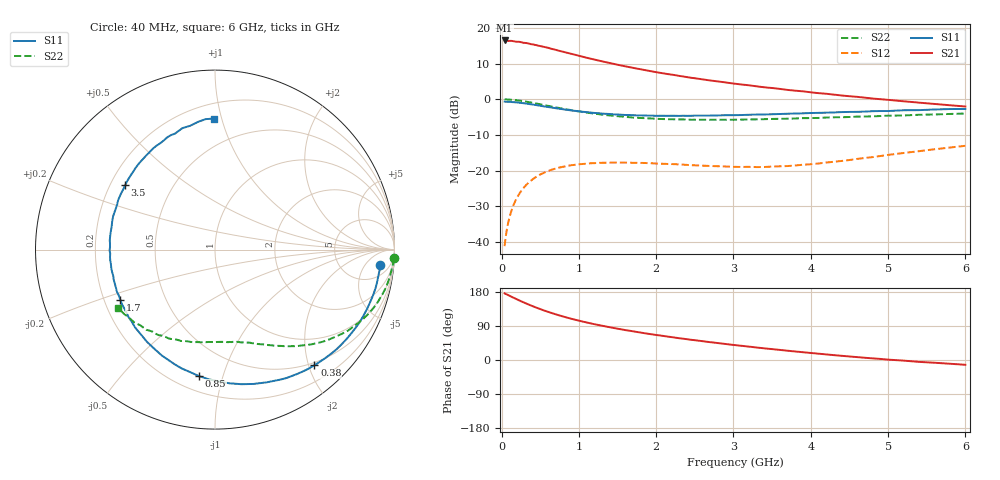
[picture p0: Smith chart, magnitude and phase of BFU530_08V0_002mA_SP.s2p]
! Filename:  P:\Prog\Test\Noise\ATS_data\Testdata_Net\03 Spar\BFU530_APG2013_40_A05_08p0V_002mA_SP_CM01_D.s2p
! Date/Time: Fri 26/Apr/2013 13:03:14
! BFU530_APG2013_40_A05_08p0V_1to25mA_SP_CM01_Bias2_R.s2p
! MDIF S-parameter v. bias file
! BFU530_APG2013_40_A05_08p0V_1to25mA_SP_CM01
! Date/time Wed Apr 24 16:58:28 2013
! VAR V_out= 8.0000
! VAR I_out= 1.9900
! VAR V_in= 0.7959
! VAR I_in= 0.0207
! Device data file deembeded for feedlines and parallel
! Original file: \03 Spar\BFU530_APG2013_40_A05_08p0V_002mA_SP_CM01_R.s2p
! Feed-files: PR047V01_250413_Feed1.s2p, PR047V01_250413_Feed2.s2p
! Parallel-file: PR047V01_250413_Par.s2p
# MHz S MA R 50
!  Freq-MHz  S11-mag  S11-arg  S21-mag  S21-arg  S12-mag  S12-arg  S22-mag  S22-arg
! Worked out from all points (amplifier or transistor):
!   98 points, 40 MHz to 6 GHz, reference 50 ohm
!   highest |S21| = 16.5 dB at 40 MHz (marker M1)
!   |S21| within 3 dB of that: start of sweep to 763.9 MHz
!   unconditionally stable (mu >= 1): 2.894 GHz to 4.763 GHz
!   at 300 MHz: K = 0.11, MSG = 20.1 dB, |S12| = -24.5 dB
!   at 1.6 GHz: K = 0.54, MSG = 13.5 dB, |S12| = -17.8 dB
!   at 6 GHz: K = 0.80, MSG = 5.5 dB, |S12| = -13.1 dB
!   S11 on the Smith chart (normalised r, x): 40 MHz: 10, -13; 380 MHz: 0.45, -2.10; 850 MHz: 0.29, -0.84; 1.7 GHz: 0.27, -0.23; 3.5 GHz: 0.26, +0.30; 6 GHz: 0.30, +0.94
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40  0.9255 -5.5  6.669 175.9  0.008713 86.6  0.9958 -2.9
50  0.9245 -6.8  6.667 174.5  0.0108 86.0  0.9954 -3.6
70  0.9218 -9.3  6.628 172.9  0.01507 84.1  0.9926 -5.3
120  0.9167 -16.2  6.591 167.8  0.02557 80.0  0.9848 -9.0
240  0.8904 -32.0  6.353 156.2  0.0491 70.5  0.9537 -17.7
320  0.868 -42.2  6.143 149.0  0.06293 64.6  0.9245 -23.1
380  0.8498 -49.3  5.919 143.9  0.07216 60.5  0.8997 -26.8
460  0.824 -58.7  5.7 137.5  0.08327 55.6  0.8684 -31.3
600  0.7787 -74.0  5.27 127.2  0.09837 47.8  0.8086 -38.3
750  0.7348 -88.4  4.76 117.6  0.1103 40.8  0.7526 -44.5
850  0.7099 -97.3  4.473 111.7  0.116 36.9  0.7181 -48.1
1050  0.667 -113.2  3.944 101.4  0.1237 30.2  0.6606 -54.5
1200  0.6431 -123.7  3.603 94.5  0.1271 26.2  0.6273 -58.5
1350  0.6248 -133.0  3.307 88.4  0.1288 23.0  0.5997 -62.0
1700  0.5973 -151.9  2.757 75.8  0.1284 17.6  0.5537 -69.5
2050  0.5868 -167.8  2.345 64.7  0.1248 14.4  0.5291 -76.3
2500  0.5887 175.1  1.97 52.2  0.1186 13.6  0.5164 -84.6
3100  0.6003 155.2  1.611 37.5  0.1124 18.2  0.5184 -95.6
3500  0.6157 144.4  1.437 28.7  0.1138 23.6  0.5294 -102.9
4100  0.6445 128.7  1.217 16.6  0.1257 31.6  0.547 -114.2
5200  0.7008 105.0  0.9362 -1.6  0.1763 36.9  0.5925 -134.6
6000  0.73 90.5  0.7911 -12.6  0.2224 33.4  0.6305 -149.2
